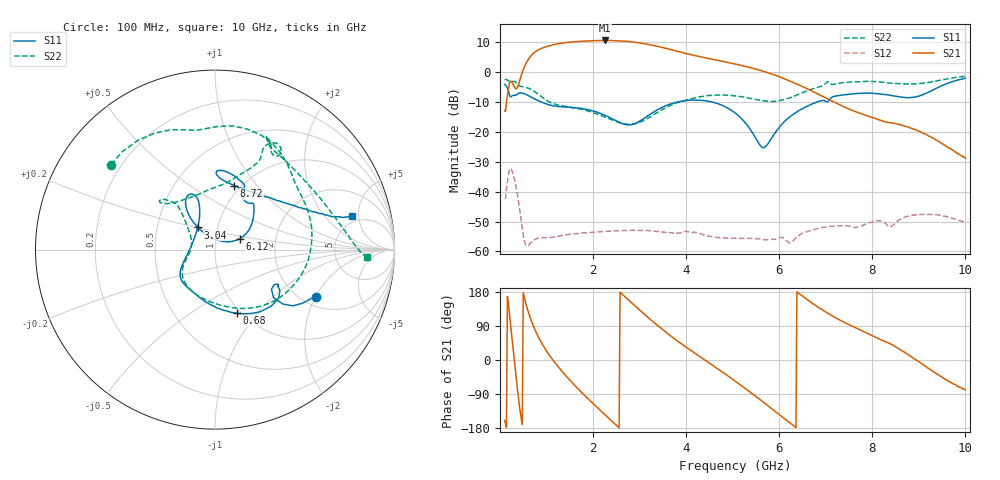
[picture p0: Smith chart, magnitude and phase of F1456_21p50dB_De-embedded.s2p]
! Integrated Device Technology
! Corporate Headquarters
! 6024 Silver Creek Valley Road
! San Jose, CA 95138  USA
! Phone:  1-408-284-8200
! Toll Free:  1-800-223-1366
! Webpage:  http://www.idt.com/
! Timing and RF Division
! 515 Groton Road, Suite 102
! Westford, MA 01886-6024
! Device:  F1456
! Description: 6-bit 0.5 dB Transmit Variable Gain Amplifier
! Frequency:  2100.0 -  2950.00 MHz
! Package:  6x6 mm Thin QFN Plastic Package: 28 pin
! State:  43
! Atten State:  21.5 dB
! Voltage:  +5.00 Volts
! Current:  216.966 mA
! Data:  The device was measured on a the F1455 evaluation board which has
!  individual transmission lines to the RF pins.  Data was collected
!  using a calibrated network analyzer.  The evaluation board was
!  de-embedded using a TRL calibration technique.
!  The reference plane is the edge of the package pin.
!  Pin  1 = CSb
!  Pin  2 = DATA
!  Pin  3 = CLK
!  Pin  4 = RSET
!  Pin  5 = GND
!  Pin  6 = RFIN  = Port 1
!  Pin  7 = GND
!  Pin  8 = NC
!  Pin  9 = NC
!  Pin 10 = NC
!  Pin 11 = NC
!  Pin 12 = NC
!  Pin 13 = NC
!  Pin 14 = /STBY
!  Pin 15 = GND
!  Pin 16 = RFOUT  = Port 2
!  Pin 17 = GND
!  Pin 18 = NC
!  Pin 19 = NC
!  Pin 20 = NC
!  Pin 21 = GND
!  Pin 22 = NC
!  Pin 23 = GND
!  Pin 24 = NC
!  Pin 25 = NC
!  Pin 26 = NC
!  Pin 27 = GND
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# GHz S dB R 50
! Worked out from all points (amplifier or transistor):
!   496 points, 100 MHz to 10 GHz, reference 50 ohm
!   highest |S21| = 10.5 dB at 2.26 GHz (marker M1)
!   |S21| within 3 dB of that: 841.4 MHz to 3.657 GHz (2.816 GHz wide, 125 % of centre)
!   unconditionally stable (mu >= 1): start of sweep to end of sweep
!   at 1.74 GHz: K = 67.44, MAG = 10.8 dB, |S12| = -53.9 dB
!   at 5.06 GHz: K = 179.72, MAG = 3.5 dB, |S12| = -55.6 dB
!   at 10 GHz: K = 500.73, MAG = -19.3 dB, |S12| = -50.3 dB
!   S11 on the Smith chart (normalised r, x): 100 MHz: 2.36, -2.01; 680 MHz: 0.96, -0.79; 3.04 GHz: 0.80, +0.20; 6.12 GHz: 1.31, +0.16; 8.72 GHz: 0.93, +0.77; 10 GHz: 4.20, +4.07
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0.1  -4.15 -25.0  -12.93 -159.6  -42.30 49.4  -2.53 140.8
0.24  -8.34 -30.8  -3.10 78.4  -32.38 -75.8  -3.40 94.4
0.32  -7.82 -30.3  -5.27 -11.7  -36.48 -152.9  -3.27 67.6
0.42  -7.04 -37.3  -3.12 -123.4  -45.68 141.5  -4.67 41.0
0.54  -7.37 -54.0  2.23 156.6  -57.45 136.3  -5.11 16.6
0.68  -8.50 -70.8  5.63 101.7  -56.84 145.9  -5.96 -15.1
0.86  -9.87 -89.5  7.65 52.6  -55.42 113.2  -7.91 -52.0
1.16  -11.37 -114.5  9.11 -3.5  -55.19 77.6  -10.65 -94.3
1.48  -11.79 -132.0  9.92 -50.5  -54.32 53.9  -11.73 -123.5
1.76  -12.22 -142.3  10.25 -86.3  -53.83 37.8  -12.54 -139.8
2.26  -14.52 -158.4  10.51 -144.8  -53.29 14.9  -15.12 -159.5
2.62  -17.25 176.1  10.36 174.3  -53.07 -0.7  -17.24 -176.7
3.04  -16.09 128.1  9.61 127.4  -52.99 -20.2  -16.55 154.1
3.4  -12.53 111.1  8.49 89.7  -53.30 -36.8  -13.39 137.9
4.12  -9.43 113.7  5.69 23.8  -53.80 -69.3  -8.93 132.0
5.06  -13.79 128.2  2.62 -56.2  -55.59 -114.7  -8.02 139.1
5.66  -25.31 72.9  0.21 -111.5  -56.08 -153.4  -9.66 122.3
6.12  -16.46 23.8  -2.38 -155.7  -55.85 173.9  -9.13 88.8
6.7  -10.76 42.1  -6.37 150.8  -52.85 150.4  -5.76 65.2
8.36  -7.75 87.8  -16.92 44.2  -51.73 73.6  -3.71 62.3
8.72  -8.60 73.3  -18.20 18.1  -48.48 70.7  -4.01 50.1
10  -2.11 13.8  -28.87 -78.4  -50.32 -21.5  -1.46 -2.6
